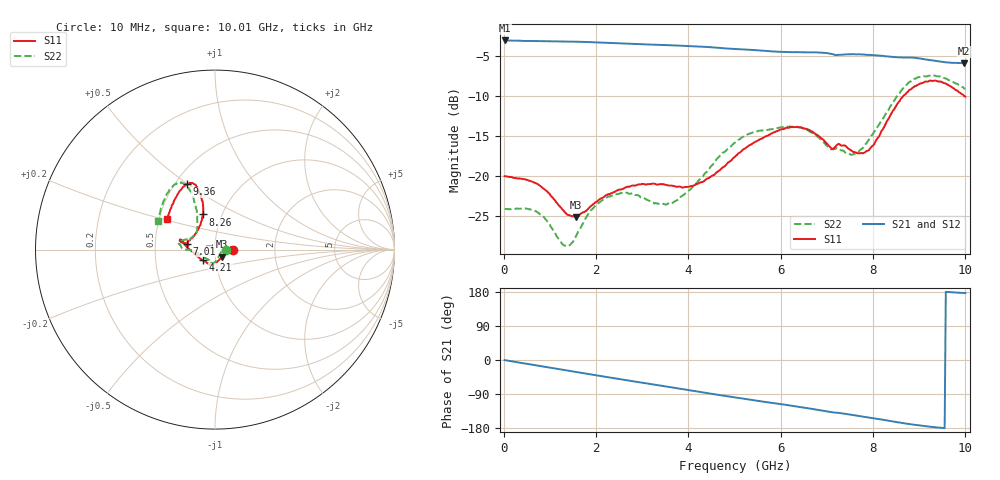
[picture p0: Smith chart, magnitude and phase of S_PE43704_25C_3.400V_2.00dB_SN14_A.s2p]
! Device ID: PE43704
! Dir: z:\PE43704\PE43704_Char_1_20130516\PE43704\AMB\3p400V\2p00dB
! Serial: 14
! Insertion: A
! Impedance: 50 ohm
! Temp: Amb
! VDD: 3.400V
! Attenuation Step: 2.00dB
! IDD: 1.139853e-01mA
#  Hz  S  RI  R  50
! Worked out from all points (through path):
!   401 points, 10 MHz to 10.01 GHz, reference 50 ohm
!   highest |S21| = -3.00 dB at 10 MHz (marker M1); lowest = -5.8 dB at 9.985 GHz (marker M2)
!   group delay of S21, straight-line fit = 52.2 ps
!   lowest |S11| = -25.1 dB at 1.56 GHz (marker M3), VSWR 1.12, Z = 53.9 - j4.31 ohm
!   |S11| at or under -10 dB: start of sweep to 8.654 GHz; 9.998769 GHz to end of sweep
!   |S22| runs from -28.7 to -7.4 dB; largest |S21 - S12| = 0.0046
!   S11 on the Smith chart (normalised r, x): 10 MHz: 1.22, +0.00; 4.21 GHz: 0.87, -0.10; 7.01 GHz: 0.73, +0.05; 8.26 GHz: 0.81, +0.33; 9.36 GHz: 0.57, +0.49; 10.01 GHz: 0.55, +0.21
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1e7  0.1002 5.74e-05  0.7083 -0.00293  0.7084 -0.00262  0.0625 0.000367
7.1e8  0.089 0.0132  0.6801 -0.1747  0.6801 -0.1746  0.0571 0.0184
1.31e9  0.0566 -0.0201  0.6246 -0.3118  0.6248 -0.3117  0.034 -0.0145
1.56e9  0.0388 -0.0399  0.5929 -0.3641  0.5927 -0.3641  0.0223 -0.0357
1.685e9  0.0305 -0.0504  0.5748 -0.3893  0.5748 -0.3892  0.0156 -0.0467
2.01e9  0.0111 -0.0686  0.5229 -0.4485  0.5231 -0.448  0.00279 -0.067
2.41e9  -0.0076 -0.08  0.4515 -0.5108  0.4518 -0.5104  -0.0117 -0.0763
3.36e9  -0.0281 -0.0847  0.2605 -0.6116  0.2612 -0.6111  -0.0288 -0.0608
3.735e9  -0.0413 -0.0757  0.1793 -0.6339  0.1802 -0.6338  -0.0508 -0.049
4.21e9  -0.0671 -0.06  0.0744 -0.6445  0.0746 -0.6443  -0.0895 -0.0259
5.01e9  -0.1328 -0.00645  -0.0947 -0.6196  -0.0943 -0.6197  -0.1628 -0.000468
6.035e9  -0.1901 0.0543  -0.2715 -0.5352  -0.2699 -0.5362  -0.2008 0.0311
6.685e9  -0.1866 0.041  -0.3765 -0.4632  -0.3769 -0.4627  -0.18 0.0518
7.01e9  -0.1559 0.034  -0.423 -0.4123  -0.4229 -0.4122  -0.1441 0.0573
7.635e9  -0.1216 0.0714  -0.4839 -0.3203  -0.4836 -0.3205  -0.1035 0.0931
7.935e9  -0.0909 0.1174  -0.5093 -0.2679  -0.5097 -0.2693  -0.0991 0.1423
8.26e9  -0.0663 0.1961  -0.5251 -0.2068  -0.5228 -0.2102  -0.1012 0.2176
8.36e9  -0.0652 0.2251  -0.5286 -0.1874  -0.5281 -0.1895  -0.1074 0.2446
8.835e9  -0.0953 0.3385  -0.5441 -0.0972  -0.5417 -0.0989  -0.1628 0.3587
9.36e9  -0.1583 0.3644  -0.5277 -0.0225  -0.5283 -0.0209  -0.2306 0.3583
9.985e9  -0.261 0.181  -0.5101 0.0286  -0.5113 0.0302  -0.3125 0.1676
1.001e10  -0.266 0.169  -0.5118 0.0294  -0.5143 0.0307  -0.3159 0.1583
